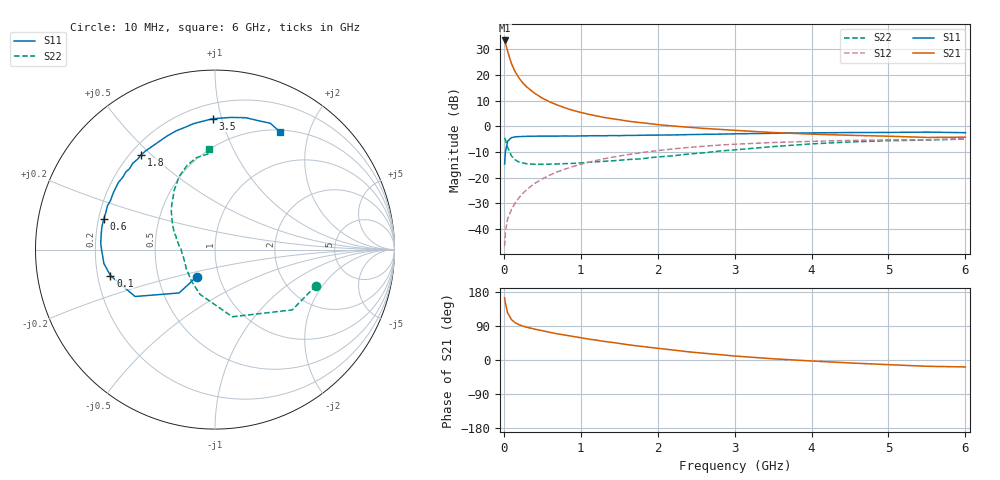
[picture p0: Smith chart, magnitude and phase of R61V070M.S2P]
! SIEMENS Small Signal Semiconductors
! BFR193
! Si NPN RF Bipolar Junction Transistor in SOT23
! VCE = 1 V  IC = 70 mA
! Common Emitter S-Parameters:  May  1996
# GHz  S  MA  R  50
!  f  S11  S21  S12  S22
! GHz  MAG  ANG  MAG  ANG  MAG  ANG  MAG  ANG
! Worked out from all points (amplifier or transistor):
!   36 points, 10 MHz to 6 GHz, reference 50 ohm
!   highest |S21| = 33.5 dB at 10 MHz (marker M1)
!   |S21| within 3 dB of that: start of sweep to 38.56 MHz
!   unconditionally stable (mu >= 1): start of sweep to 16.88 MHz; 142 MHz to end of sweep
!   at 250 MHz: K = 1.09, MAG = 19.6 dB, |S12| = -26.1 dB
!   at 1.4 GHz: K = 1.08, MAG = 5.8 dB, |S12| = -12.1 dB
!   at 6 GHz: K = 1.02, MAG = -0.6 dB, |S12| = -4.8 dB
!   S11 on the Smith chart (normalised r, x): 10 MHz: 0.78, -0.25; 100 MHz: 0.25, -0.12; 600 MHz: 0.22, +0.13; 1.8 GHz: 0.24, +0.46; 3.5 GHz: 0.30, +0.94; 6 GHz: 0.52, +1.56
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0.01  0.1836 -124.1  47.06 164.0  0.0046 66.2  0.5976 -19.6
0.02  0.3135 -129.6  42.73 150.1  0.0087 66.0  0.5458 -38.0
0.05  0.5164 -149.6  28.58 124.1  0.0159 62.0  0.3865 -75.5
0.1  0.6003 -166.0  16.45 106.4  0.024 64.0  0.2629 -108.5
0.15  0.6239 -172.9  11.38 98.1  0.0324 68.2  0.2197 -126.6
0.2  0.6278 -177.3  8.615 93.0  0.0409 70.7  0.1996 -138.0
0.25  0.6334 179.3  6.897 89.2  0.0497 71.9  0.1917 -146.9
0.3  0.6374 177.1  5.798 86.4  0.0588 72.4  0.1859 -152.0
0.4  0.6402 171.7  4.406 81.5  0.0766 72.7  0.1816 -160.3
0.5  0.6429 168.6  3.531 77.3  0.0942 72.1  0.181 -166.7
0.6  0.6428 164.7  2.967 73.0  0.112 71.2  0.1825 -170.7
0.7  0.6424 161.1  2.578 68.9  0.1299 70.0  0.1843 -173.9
0.8  0.6471 157.8  2.272 65.6  0.147 68.3  0.1871 -177.1
0.9  0.6432 154.9  2.04 62.1  0.1645 66.8  0.1888 179.6
1.1  0.6512 148.3  1.716 55.3  0.1986 63.4  0.1985 175.3
1.3  0.6527 141.9  1.489 49.1  0.2318 59.8  0.2074 170.3
1.8  0.6688 128.1  1.167 35.8  0.3081 50.6  0.2334 160.2
2.2  0.677 117.9  1.011 26.3  0.3619 43.3  0.2658 151.6
3.5  0.7296 90.9  0.755 3.2  0.4821 20.5  0.4017 124.4
4.5  0.7546 76.8  0.667 -7.8  0.5297 6.6  0.4944 108.3
5.5  0.7686 66.4  0.606 -16.6  0.5459 -5.9  0.5381 92.7
6  0.7496 61.3  0.613 -18.3  0.5734 -9.7  0.5636 93.5
